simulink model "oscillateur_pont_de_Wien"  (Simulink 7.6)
settings: Solver=ode23tb  StartTime=0.0  StopTime=0.5  RelTol=1e-3
InitFcn:
  | R=1e3;
  | R1=10e3;
  | R2=22e3;
  | C=1e-6;
StopFcn:
  | close all
  | load oscillateur_pont_de_Wien.mat
  | plot(x(1,:),x(2,:))
  | hold on
  | grid
  | title('Oscillateur à pont de Wien')
  | xlabel('temps')
  | delete *.mat
libraries: powerlib x20

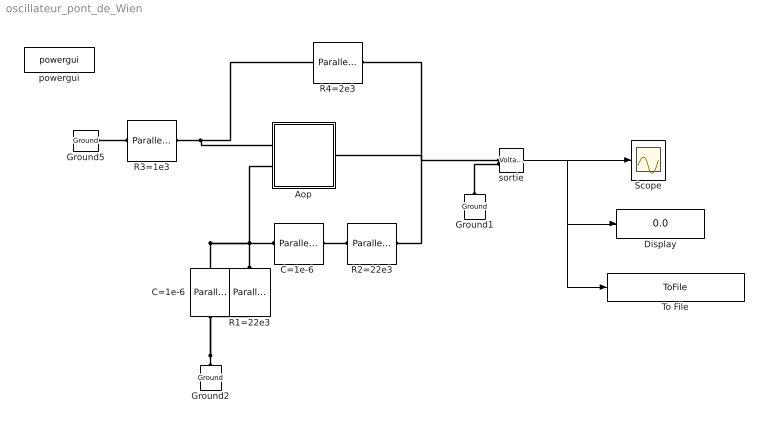
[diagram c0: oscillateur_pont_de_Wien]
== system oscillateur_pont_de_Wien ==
  Aop : Subsystem
  C=1e-6 : powerlib/Elements/Parallel RLC Branch  DialogController=POWERSYS.PowerSysDialog  PhysicalDomain=powersysdomain  SubClassName=unknown  LeftPortType=p1  RightPortType=p1  LConnTagsString=a  RConnTagsString=__new0  BranchType=C  Resistance=R  Inductance=10e-03  SetiL0=off  InitialCurrent=0  Capacitance=C  Setx0=on  InitialVoltage=6  Measurements=None
  "C=1e-6 " : powerlib/Elements/Parallel RLC Branch  DialogController=POWERSYS.PowerSysDialog  PhysicalDomain=powersysdomain  SubClassName=unknown  LeftPortType=p1  RightPortType=p1  LConnTagsString=a  RConnTagsString=__new0  BranchType=C  Resistance=R  Inductance=10e-03  SetiL0=off  InitialCurrent=0  Capacitance=C  Setx0=off  InitialVoltage=0  Measurements=None
  Display : Display
  Ground1 : powerlib/Elements/Ground  DialogController=POWERSYS.PowerSysDialog  PhysicalDomain=powersysdomain  SubClassName=unknown  LeftPortType=p1  RightPortType=p1  LConnTagsString=a
  Ground2 : powerlib/Elements/Ground  DialogController=POWERSYS.PowerSysDialog  PhysicalDomain=powersysdomain  SubClassName=unknown  LeftPortType=p1  RightPortType=p1  LConnTagsString=a
  Ground5 : powerlib/Elements/Ground  DialogController=POWERSYS.PowerSysDialog  PhysicalDomain=powersysdomain  SubClassName=unknown  LeftPortType=p1  RightPortType=p1  LConnTagsString=a
  R1=22e3 : powerlib/Elements/Parallel RLC Branch  DialogController=POWERSYS.PowerSysDialog  PhysicalDomain=powersysdomain  SubClassName=unknown  LeftPortType=p1  RightPortType=p1  LConnTagsString=a  RConnTagsString=__new0  BranchType=R  Resistance=R2  Inductance=10e-03  SetiL0=off  InitialCurrent=0  Capacitance=[]  Setx0=off  InitialVoltage=0  Measurements=None
  R2=22e3 : powerlib/Elements/Parallel RLC Branch  DialogController=POWERSYS.PowerSysDialog  PhysicalDomain=powersysdomain  SubClassName=unknown  LeftPortType=p1  RightPortType=p1  LConnTagsString=a  RConnTagsString=__new0  BranchType=R  Resistance=R2  Inductance=10e-03  SetiL0=off  InitialCurrent=0  Capacitance=[]  Setx0=off  InitialVoltage=0  Measurements=None
  R3=1e3 : powerlib/Elements/Parallel RLC Branch  DialogController=POWERSYS.PowerSysDialog  PhysicalDomain=powersysdomain  SubClassName=unknown  LeftPortType=p1  RightPortType=p1  LConnTagsString=a  RConnTagsString=__new0  BranchType=R  Resistance=R  Inductance=10e-03  SetiL0=off  InitialCurrent=0  Capacitance=[]  Setx0=off  InitialVoltage=0  Measurements=None
  R4=2e3 : powerlib/Elements/Parallel RLC Branch  DialogController=POWERSYS.PowerSysDialog  PhysicalDomain=powersysdomain  SubClassName=unknown  LeftPortType=p1  RightPortType=p1  LConnTagsString=a  RConnTagsString=__new0  BranchType=R  Resistance=2*R  Inductance=10e-03  SetiL0=off  InitialCurrent=0  Capacitance=[]  Setx0=off  InitialVoltage=0  Measurements=None
  Scope : Scope
  To File : ToFile  Filename=oscillateur_pont_de_Wien  MatrixName=x
  powergui : powerlib/powergui  SystemSampleTime=-1  SimulationMode=Continuous  SampleTime=0  frequency=60  SPID=off  DisableSnubberDevices=off  DisableRonSwitches=off  DisableVfSwitches=off  SwTol=0  Interpol=off  frequencyindice=0  echomessages=off  HookPort=off  DisplayEquations=off  FunctionMessages=off  EnableUseOfTLC=off  x0status=blocks  RestoreLinks=warning  ResistiveCurrentMeasurement=off  Frange=[0:2:500]  Ylog=off  Xlog=on  ShowGrid=off  save=off  variable=ZData  structure=ScopeData1  ZoomFFT=off  StartTime=0.0  cycles=1  DisplayStyle=1  fundamental=10  FreqAxis=off  MaxFrequency=100  frequencyindicesteady=60  RmsSteady=1  display=off  Ts=0  methode=off
  sortie : powerlib/Measurements/Voltage Measurement  DialogController=POWERSYS.PowerSysDialog  SystemSampleTime=-1  PhasorSimulation=off  OutputType=Complex  PSBequivalent=0
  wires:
  sortie/1 -> Scope/1, Display/1, To File/1
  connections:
  Aop/RConn1 -- sortie/LConn1 -- R4=2e3/LConn1 -- R2=22e3/LConn1
  R3=1e3/LConn1 -- R4=2e3/RConn1 -- Aop/LConn1
  Ground5/LConn1 -- R3=1e3/RConn1
  C=1e-6/LConn1 -- Aop/LConn2 -- "C=1e-6 "/LConn1 -- R1=22e3/LConn1
  "C=1e-6 "/RConn1 -- R2=22e3/RConn1
  Ground1/LConn1 -- sortie/LConn2
  Ground2/LConn1 -- C=1e-6/RConn1 -- R1=22e3/RConn1

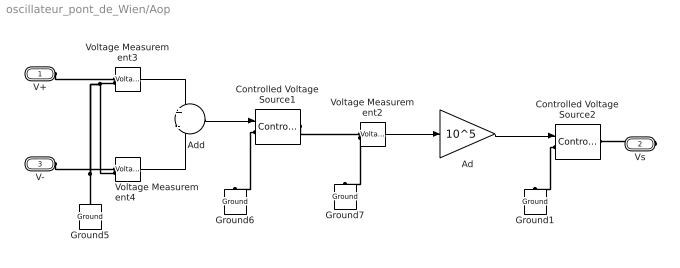
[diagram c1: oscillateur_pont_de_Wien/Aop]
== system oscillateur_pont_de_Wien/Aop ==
  Ad : Gain  Gain=10^5
  Add : Sum  Inputs=+-
  Controlled Voltage Source1 : powerlib/Electrical Sources/Controlled Voltage Source  DialogController=POWERSYS.PowerSysDialog  SystemSampleTime=-1  Initialize=on  Source_Type=AC  Amplitude=0  Phase=0  Frequency=0  Measurements=None
  Controlled Voltage Source2 : powerlib/Electrical Sources/Controlled Voltage Source  DialogController=POWERSYS.PowerSysDialog  SystemSampleTime=-1  Initialize=on  Source_Type=AC  Amplitude=0  Phase=0  Frequency=0  Measurements=None
  Ground{1,5..7} (4 alike) : powerlib/Elements/Ground  DialogController=POWERSYS.PowerSysDialog  PhysicalDomain=powersysdomain  SubClassName=unknown  LeftPortType=p1  RightPortType=p1  LConnTagsString=a
  Voltage Measurement2 : powerlib/Measurements/Voltage Measurement  DialogController=POWERSYS.PowerSysDialog  SystemSampleTime=-1  PhasorSimulation=off  OutputType=Complex  PSBequivalent=0
  Voltage Measurement3 : powerlib/Measurements/Voltage Measurement  DialogController=POWERSYS.PowerSysDialog  SystemSampleTime=-1  PhasorSimulation=off  OutputType=Complex  PSBequivalent=0
  Voltage Measurement4 : powerlib/Measurements/Voltage Measurement  DialogController=POWERSYS.PowerSysDialog  SystemSampleTime=-1  PhasorSimulation=off  OutputType=Complex  PSBequivalent=0
  V+ : PMIOPort  Port=1  Side=Left
  Vs : PMIOPort  Port=2  Side=Right
  V- : PMIOPort  Port=3  Side=Left
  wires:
  Add/1 -> Controlled Voltage Source1/1
  Voltage Measurement2/1 -> Ad/1
  Voltage Measurement4/1 -> Add/2
  Voltage Measurement3/1 -> Add/1
  Ad/1 -> Controlled Voltage Source2/1
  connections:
  Controlled Voltage Source1/LConn1 -- Ground6/LConn1
  Controlled Voltage Source1/RConn1 -- Voltage Measurement2/LConn1
  Controlled Voltage Source2/LConn1 -- Ground1/LConn1
  Voltage Measurement3/LConn2 -- Voltage Measurement4/LConn2 -- Ground5/LConn1
  Voltage Measurement2/LConn2 -- Ground7/LConn1
  V+/RConn1 -- Voltage Measurement3/LConn1
  Vs/RConn1 -- Controlled Voltage Source2/RConn1
  V-/RConn1 -- Voltage Measurement4/LConn1
